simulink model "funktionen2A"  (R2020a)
settings: Solver=ode45  StartTime=0.0  StopTime=10.0  MaxStep=1e-2  RelTol=1e-3  EnableMultiTasking=on
libraries: simulink x1

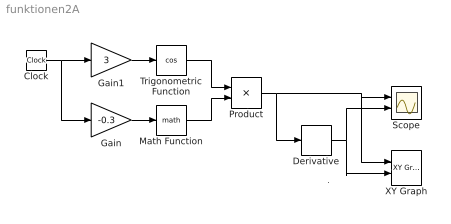
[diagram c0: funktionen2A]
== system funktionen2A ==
  note: .
  Clock : Clock
  Derivative : Derivative
  Gain : Gain  Gain=-0.3  SaturateOnIntegerOverflow=on
  Gain1 : Gain  Gain=3  SaturateOnIntegerOverflow=on
  Math Function : Math  SignedPower=on
  Product : Product  SaturateOnIntegerOverflow=on
  Scope : Scope  NumInputPorts=2
  Trigonometric Function : Trigonometry  Operator=cos
  XY Graph : simulink/Sinks/XY Graph  xmin=-1  xmax=1  ymin=-2.7  ymax=2.7  st=-1
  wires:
  Clock/1 -> Gain/1, Gain1/1
  Product/1 -> Derivative/1, Scope/1, XY Graph/1
  Derivative/1 -> Scope/2, XY Graph/2
  Gain/1 -> Math Function/1
  Trigonometric Function/1 -> Product/1
  Math Function/1 -> Product/2
  Gain1/1 -> Trigonometric Function/1
